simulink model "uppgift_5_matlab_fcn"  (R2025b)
settings: Solver=VariableStepAuto  StartTime=0.0  StopTime=10.0  RelTol=1e-3
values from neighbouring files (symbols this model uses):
  tau_d = 0.2    [Lektion_2.m]
  tau_mix = 0.14    [Lektion_2.m]
  tau_sensor = 0.05    [Lektion_2.m]

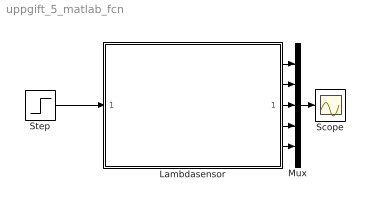
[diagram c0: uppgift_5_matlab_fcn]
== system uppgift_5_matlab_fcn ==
  Lambdasensor : Subsystem
  Mux : Mux  Inputs=5
  Scope : Scope
  Step : Step  Time=5  Before=0.8  After=1.2  SampleTime=0
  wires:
  Lambdasensor/1(lambda_cyl [-]) -> Mux/1
  Lambdasensor/2(lambda_delay [-]) -> Mux/2
  Lambdasensor/3(lambda_eg [-]) -> Mux/3
  Lambdasensor/4(lambda_sensor [-]) -> Mux/4
  Lambdasensor/5(lambda_d [-]) -> Mux/5
  Mux/1 -> Scope/1
  Step/1 -> Lambdasensor/1(lambda_c [-])

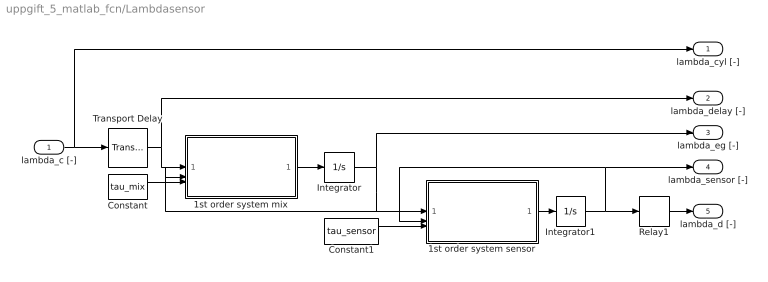
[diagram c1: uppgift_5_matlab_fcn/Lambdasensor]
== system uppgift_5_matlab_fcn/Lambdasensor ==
  lambda_c [-] : Inport
  1st order system mix : MATLAB Function  TreatAsAtomicUnit=on
  1st order system sensor : MATLAB Function  TreatAsAtomicUnit=on
  Constant : Constant  Value=tau_mix
  Constant1 : Constant  Value=tau_sensor
  Integrator : Integrator  InitialCondition=0.8
  Integrator1 : Integrator  InitialCondition=0.8
  Relay1 : Relay  OnSwitchValue=1+eps  OffSwitchValue=1-eps
  Transport Delay : TransportDelay  DelayTime=tau_d  InitialOutput=0.8
  lambda_cyl [-] : Outport
  lambda_delay [-] : Outport  Port=2
  lambda_eg [-] : Outport  Port=3
  lambda_sensor [-] : Outport  Port=4
  lambda_d [-] : Outport  Port=5
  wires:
  lambda_c [-]/1 -> lambda_cyl [-]/1, Transport Delay/1
  Transport Delay/1 -> 1st order system mix/1(ref), lambda_delay [-]/1
  1st order system mix/1(alpha) -> Integrator/1
  Integrator/1 -> 1st order system sensor/1(ref), 1st order system mix/2(actual), lambda_eg [-]/1
  Integrator1/1 -> 1st order system sensor/2(actual), lambda_sensor [-]/1, Relay1/1
  Relay1/1 -> lambda_d [-]/1
  Constant/1 -> 1st order system mix/3(tau)
  Constant1/1 -> 1st order system sensor/3(tau)
  1st order system sensor/1(alpha) -> Integrator1/1

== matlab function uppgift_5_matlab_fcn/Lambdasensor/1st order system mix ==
function alpha = fcn(ref, actual, tau)
error = ref - actual;

alpha =  error*tau;

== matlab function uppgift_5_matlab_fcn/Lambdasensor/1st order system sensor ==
function alpha = fcn(ref, actual, tau)
error = ref - actual;

alpha =  error*tau;
